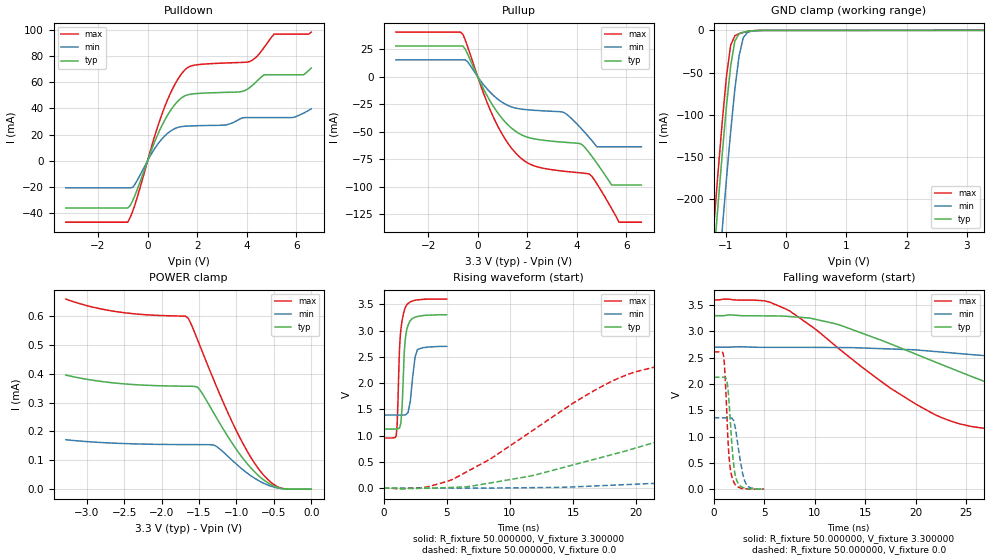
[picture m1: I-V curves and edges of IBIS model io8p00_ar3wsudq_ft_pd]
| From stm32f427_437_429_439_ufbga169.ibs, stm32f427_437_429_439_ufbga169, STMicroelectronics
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|   Model io8p00_ar3wsudq_ft_pd
[Model]  io8p00_ar3wsudq_ft_pd
Model_type I/O
Polarity   Non-Inverting
Enable   Active-Low
Vinl =   0.990000V
Vinh =   2.310000V
Vmeas =  1.650000V
Cref =   50.000000pF
Rref =   100.000000M
Vref =   0.0V
C_comp   3.843200pF   3.761700pF   3.937000pF
[Temperature Range]   25.000000   0.125000k   -40.000000
[Pullup Reference]   3.300000V   2.700000V   3.600000V
[Pulldown Reference]   0.0V   0.0V   0.0V
[POWER Clamp Reference]   3.300000V   2.700000V   3.600000V
[GND Clamp Reference]   0.0V   0.0V   0.0V
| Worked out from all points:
|   slope of the pulldown table from 0 to 0.495 V, typ, clamps not added: 20.9 ohm
|   slope of the pullup table from 0 to 0.495 V, typ, clamps not added: 22.6 ohm
|   GND clamp passes 1 mA (typ) near -0.62 V on its own axis
|   rising waveform, R_fixture 50.000000, V_fixture 3.300000: 20-80 % time 267ps typ, 349ps min, 281ps max; typ from 1.12 V to 3.3 V
|   rising waveform, R_fixture 50.000000, V_fixture 0.0: 20-80 % time 19.8ns typ, 50.7ns min, 10.4ns max; typ from 0 V to 2.13 V
|   falling waveform, R_fixture 50.000000, V_fixture 3.300000: 20-80 % time 18.5ns typ, 39.7ns min, 11.4ns max; typ from 3.3 V to 1.12 V
|   falling waveform, R_fixture 50.000000, V_fixture 0.0: 20-80 % time 504ps typ, 695ps min, 421ps max; typ from 2.13 V to 0 V
[Pulldown]
|Voltage   I(typ)   I(min)   I(max)
-3.3V     -36.18mA   -20.77mA   -47.07mA
-800mV    -36.18mA   -20.77mA   -47.07mA
-600mV    -30.5mA    -20.52mA   -38.69mA
700mV     31.4mA     19.11mA    41.71mA
1.2V      45.15mA    25.37mA    61.75mA
1.6V      50.35mA    26.5mA     71.06mA
3.1V      52.27mA    27.26mA    74.75mA
4.1V      55.7mA     33.01mA    75.8mA
4.7V      65.73mA    33.01mA    86.69mA
5.1V      65.73mA    33.01mA    96.89mA
6.3V      65.85mA    36.49mA    96.89mA
6.6V      70.9mA     39.7mA     98.44mA
[Pullup]
|Voltage   I(typ)   I(min)   I(max)
-3.3V     28.03mA    15.43mA    40.67mA
-700mV    28.03mA    15.43mA    40.67mA
-400mV    20.31mA    13.47mA    26.93mA
600mV     -25.77mA   -16.23mA   -35.13mA
1.6V      -50.64mA   -28.81mA   -70.96mA
3.5V      -59.53mA   -32.72mA   -85.92mA
4.2V      -61.52mA   -47.62mA   -87.46mA
4.5V      -69.21mA   -55.27mA   -88.44mA
4.8V      -78.37mA   -63.6mA    -97.02mA
5.4V      -98.4mA    -63.6mA    -119.7mA
5.7V      -98.4mA    -63.6mA    -132.2mA
6.6V      -98.4mA    -63.6mA    -132.2mA
[GND_clamp]
|Voltage   I(typ)   I(min)   I(max)
-3.3V     -2.327A    -2.405A    -2.301A
-1.2V     -270.2mA   -361.4mA   -232.1mA
-1.13V    -207.3mA   -298.1mA   -169mA
-1.06V    -146.7mA   -236.2mA   -108.8mA
-990mV    -90.18mA   -176.4mA   -54.97mA
-920mV    -42.21mA   -120mA     -17.69mA
-850mV    -12.58mA   -69.47mA   -6.279mA
-780mV    -3.983mA   -30.01mA   -3.9mA
-710mV    -2.112mA   -8.623mA   -2.396mA
-640mV    -1.159mA   -2.292mA   -1.234mA
-570mV    -535.1uA   -830.5uA   -490.2uA
3.28V     81.28uA    57.87uA    93.98uA
[POWER_clamp]
|Voltage   I(typ)   I(min)   I(max)
-3.28V    395.3uA    171.3uA    658.7uA
-2.6V     367.1uA    159uA      614.9uA
-1.68V    356.7uA    154.4uA    599.4uA
-1.64V    356.5uA    154.4uA    590.8uA
-1.52V    353.6uA    154.3uA    518.3uA
-1.48V    341.1uA    154.2uA    492.3uA
-1.28V    253.6uA    150.4uA    364.2uA
-960mV    123.1uA    77.56uA    181.6uA
-720mV    50.52uA    32.03uA    76.18uA
-560mV    18.94uA    12.27uA    28.65uA
-440mV    5.104uA    3.69uA     7.327uA
0V        0A         0A         0A
[Ramp]
| variable   typ   min   max
dV/dt_r  1.27674/19.73534n   0.81528/50.79357n   1.56654/10.33649n
dV/dt_f  1.30698/18.53201n   0.78492/39.79351n   1.58742/11.39464n
R_load = 50.000000
[Rising Waveform]
R_fixture= 50.000000
V_fixture= 3.300000
V_fixture_min= 2.700000
V_fixture_max= 3.600000
|time   V(typ)   V(min)   V(max)
0s        1.123V     1.39V      953.1mV
1.001ns   1.125V     1.391V     1.007V
1.071ns   1.127V     1.391V     1.223V
1.331ns   1.207V     1.39V      2.934V
1.461ns   1.552V     1.39V      3.187V
1.632ns   2.574V     1.392V     3.377V
1.732ns   2.868V     1.396V     3.446V
2.112ns   3.186V     1.654V     3.546V
2.673ns   3.266V     2.636V     3.583V
4.985ns   3.299V     2.699V     3.599V
[Rising Waveform]
R_fixture= 50.000000
V_fixture= 0.0
V_fixture_min= 0.0
V_fixture_max= 0.0
|time   V(typ)   V(min)   V(max)
0s        7.464nV    340.4nV    5.071nV
5.506ns   13.32mV    -138.1uV   170.5mV
11.51ns   223.8mV    7.752mV    1.049V
19.52ns   731.9mV    69.39mV    2.179V
27.03ns   1.249V     155mV      2.476V
38.04ns   1.837V     349.2mV    2.571V
57.06ns   2.064V     699.1mV    2.607V
88.09ns   2.117V     1.131V     2.611V
115.1ns   2.127V     1.291V     2.611V
249.2ns   2.128V     1.358V     2.611V
[Falling Waveform]
R_fixture= 50.000000
V_fixture= 3.300000
V_fixture_min= 2.700000
V_fixture_max= 3.600000
|time   V(typ)   V(min)   V(max)
0s        3.299V     2.699V     3.599V
5.506ns   3.295V     2.697V     3.559V
12.01ns   3.147V     2.694V     2.733V
22.02ns   2.411V     2.616V     1.407V
25.53ns   2.144V     2.56V      1.192V
31.53ns   1.723V     2.431V     1.074V
38.04ns   1.426V     2.277V     1.026V
45.55ns   1.285V     2.11V      1V
84.58ns   1.147V     1.536V     956.3mV
249.2ns   1.123V     1.39V      953.1mV
[Falling Waveform]
R_fixture= 50.000000
V_fixture= 0.0
V_fixture_min= 0.0
V_fixture_max= 0.0
|time   V(typ)   V(min)   V(max)
0s        2.128V     1.358V     2.611V
981ps     2.129V     1.357V     2.519V
1.151ns   2.12V      1.357V     2.039V
1.311ns   2.04V      1.357V     1.354V
1.502ns   1.685V     1.359V     642.8mV
1.892ns   620.5mV    1.323V     178mV
2.292ns   158.2mV    968.5mV    53.2mV
2.853ns   33.41mV    303.8mV    12.18mV
3.173ns   15.48mV    110mV      7.875mV
4.985ns   7.464nV    340.4nV    5.071nV
